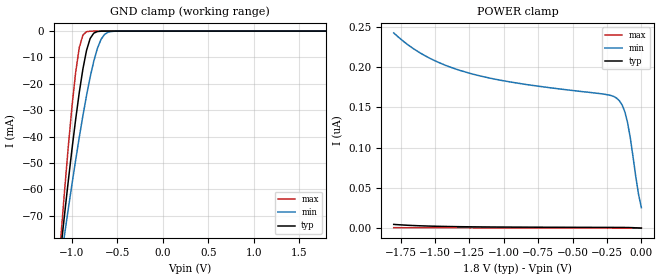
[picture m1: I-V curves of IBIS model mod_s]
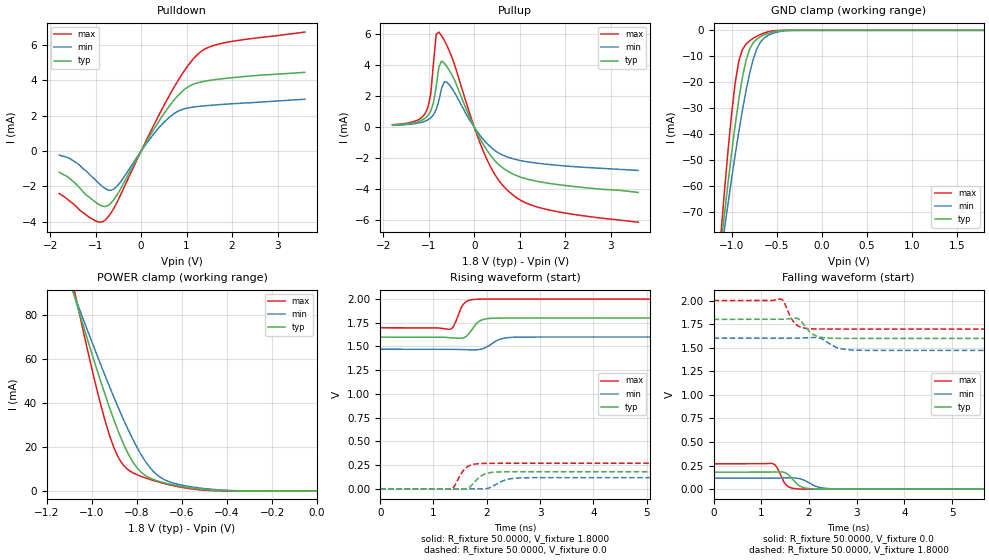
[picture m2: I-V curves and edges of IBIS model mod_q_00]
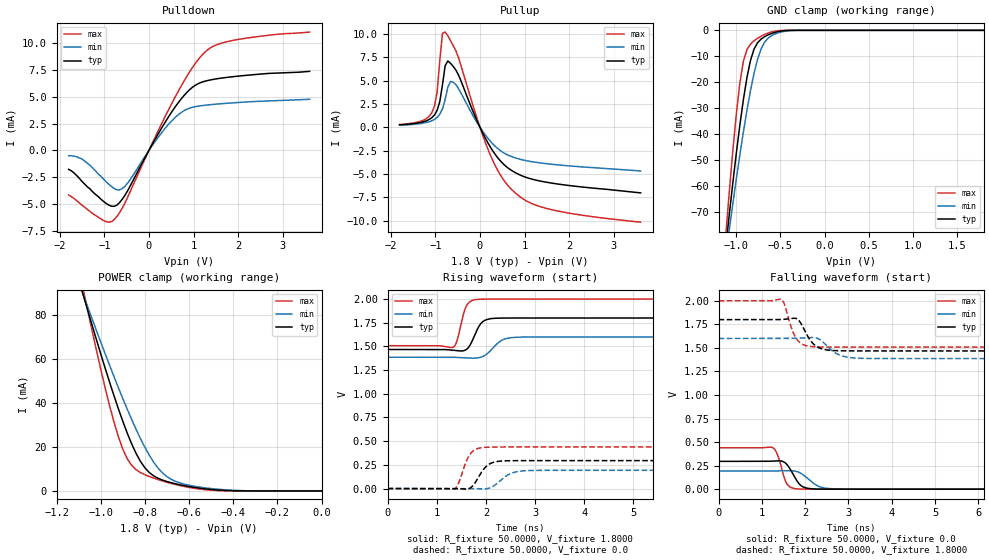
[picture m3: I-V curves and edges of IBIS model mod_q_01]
| IBIS file pin2_1v8_11.ibs created by s2ibis3 verion 1.1
| North Carolina State University, ERL, 2006
[IBIS ver]  4.0
[File name] pe_11_m95p32_1d8.ibs
[File Rev]  1.0
[Date]   18 Nov 2024
[Source]   CAD & Design Services (Catania) - STMicroelectronics
[Notes]
   (Note1)  This IBIS model includes the SO8N package parasitic data
   (Note2)  Pin 2 (S) and Pin 3,5,7 (WO2,DO0,HO3) have four driver
   stength cases: High, Medium, Qlow, Low;
   (Note3)  This IBIS model has some Notes about the non-monotonicity
   of the I-V curves, but they are not indicative of problems
   inside the model;
[Disclaimer]
   Customers are solely responsible for all aspects of their
   own product designs or applications using this IBIS Model.
   STMicroelectronics assumes no liability for Custmer Designs
   and applications associated to this IBIS Model.
   In the use of this IBIS Model Customer shall not modify,
   disassemble, alter this Model in whole or in part.
   If Customers do not accept these terms, the IBIS Model
   may not be used. For any problems or modifications please
   contact STMicroelectronics (www.st.com).
[Copyright] (c) 2024 STMicroelectronics
|   Component M95P32
[Component] M95P32
[Manufacturer] STMicroelectronics
[Package]
| variable  typ   min   max
R_pkg   0.0   0.0   0.0
L_pkg   0.0H   0.0H   0.0H
C_pkg   0.0F   0.0F   0.0F
[Pin]  signal_name   model_name   R_pin   L_pin   C_pin
1   S   mod_s   129.1m   2.1741nH   1.0266pF
2   QO1   mod_q   89.7m   1.6160nH   0.3359pF
3   WO2   mod_dwh   91.2m   1.6289nH   0.3576pF
4   VSS   GND   130.9m   2.1824nH   0.2874pF
5   DO0   mod_dwh   130.7m   2.1818nH   0.2862pF
6   C   mod_c   85.3m   1.5892nH   0.3544pF
7   HO3   mod_dwh   84.5m   1.5827nH   0.3547pF
8   VDD   POWER   124.1m   2.1422nH   0.2841pF
[Model Selector]   mod_q
mod_q_11   High drive: bit0='1', bit1='1'
mod_q_10   Med drive:  bit0='1', bit1='0'
mod_q_01   Qlow drive: bit0='0', bit1='1'
mod_q_00   Low drive:  bit0='0', bit1='0'
[Model Selector]   mod_dwh
mod_dwh_11   High drive: bit0='1', bit1='1'
mod_dwh_10   Med drive:  bit0='1', bit1='0'
mod_dwh_01   Qlow drive: bit0='0', bit1='1'
mod_dwh_00   Low drive:  bit0='0', bit1='0'
| Models and submodels in the file (10): mod_s (Input), mod_q_00 (Output), mod_q_01 (Output), mod_q_10 (Output), mod_q_11 (Output), mod_c (Input), mod_dwh_00 (I/O), mod_dwh_01 (I/O), mod_dwh_10 (I/O), mod_dwh_11 (I/O)
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|   Model mod_s
[Model]   mod_s
Model_type Input
Vinl   =   0.540V
Vinh   =   1.260V
C_comp   1.014pF   0.968pF   1.062pF
[Model Spec]
Vinl   0.540V  0.480V  0.600V  | <- for Vcc = 1.8V, 1.6V, 2.0V
Vinh   1.260V  1.120V  1.400V  | <- for Vcc = 1.8V, 1.6V, 2.0V
[Temperature Range]  25.0000   0.1050k   -40.0000
[Voltage Range]   1.8000V   1.6000V   2.0000V
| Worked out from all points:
|   GND clamp passes 1 mA (typ) near -0.76 V on its own axis
[GND_clamp]
|Voltage   I(typ)   I(min)   I(max)
-1.8V     -318.6mA   -262.3mA   -406.1mA
-1.12V    -81.69mA   -86.38mA   -77.02mA
-1.08V    -68.96mA   -76.72mA   -59.82mA
-1V       -44.75mA   -57.99mA   -28.59mA
-960mV    -33.58mA   -49mA      -15.76mA
-920mV    -23.34mA   -40.35mA   -6.304mA
-880mV    -14.41mA   -32.13mA   -1.515mA
-840mV    -7.357mA   -24.45mA   -241.6uA
-800mV    -2.808mA   -17.47mA   -33.89uA
-720mV    -178.3uA   -6.536mA   -639nA
-600mV    -1.717uA   -403.8uA   -1.818nA
1.8V      181.1pA    163.5nA    12.41pA
[POWER_clamp]
|Voltage   I(typ)   I(min)   I(max)
-1.8V     4.752nA    242.5nA    716.8pA
-1.6V     2.958nA    216.8nA    597.9pA
-1.3V     1.856nA    195nA      499.1pA
-940mV    1.384nA    181.2nA    411.6pA
-280mV    1.019nA    166.7nA    267.4pA
-180mV    972.8pA    161.5nA    245.7pA
-140mV    942.2pA    153.1nA    235.1pA
-120mV    914.3pA    144.4nA    228.4pA
-100mV    866.7pA    130.9nA    219.3pA
-80mV     784.6pA    111.7nA    205.6pA
-20mV     313.3pA    41.65nA    107.7pA
0V        181.1pA    25.55nA    69.35pA
|   Model mod_q_00
[Model]   mod_q_00
Model_type Output
Polarity   Non-Inverting
Enable   Active-High
Vmeas  =   0.900V
Cref   =   30.0pF
C_comp   1.630pF   1.607pF   1.683pF
[Model Spec]
Vmeas  0.900V  0.800V  1.000V  | <- for Vcc = 1.8V, 1.6V, 2.0V
[Temperature Range]  25.0000   0.1050k   -40.0000
[Voltage Range]   1.8000V   1.6000V   2.0000V
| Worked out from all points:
|   slope of the pulldown table from 0 to 0.27 V, typ, clamps not added: 227 ohm
|   slope of the pullup table from 0 to 0.27 V, typ, clamps not added: 188 ohm
|   GND clamp passes 1 mA (typ) near -0.58 V on its own axis
|   POWER clamp passes 1 mA (typ) near -0.53 V on its own axis
|   rising waveform, R_fixture 50.0000, V_fixture 1.8000: 20-80 % time 173ps typ, 233ps min, 138ps max; typ from 1.6 V to 1.8 V
|   rising waveform, R_fixture 50.0000, V_fixture 0.0: 20-80 % time 207ps typ, 255ps min, 179ps max; typ from 0 V to 0.18 V
|   falling waveform, R_fixture 50.0000, V_fixture 0.0: 20-80 % time 213ps typ, 282ps min, 161ps max; typ from 0.18 V to 0 V
|   falling waveform, R_fixture 50.0000, V_fixture 1.8000: 20-80 % time 224ps typ, 277ps min, 188ps max; typ from 1.8 V to 1.6 V
[Pulldown]
|Voltage   I(typ)   I(min)   I(max)
-1.8V     -1.2mA     -220uA     -2.4mA
-1.38V    -2mA       -730uA     -3.26mA
-1.02V    -2.85mA    -1.59mA    -3.92mA
-840mV    -3.125mA   -2.02mA    -3.993mA
-660mV    -2.931mA   -2.218mA   -3.494mA
-540mV    -2.525mA   -2.014mA   -2.958mA
240mV     1.064mA    846.5uA    1.267mA
660mV     2.681mA    2.001mA    3.324mA
960mV     3.505mA    2.404mA    4.584mA
1.26V     3.879mA    2.53mA     5.517mA
1.86V     4.122mA    2.659mA    6.148mA
3.6V      4.46mA     2.94mA     6.74mA
[Pullup]
|Voltage   I(typ)   I(min)   I(max)
-1.8V     160uA      130uA      180uA
-1.08V    602uA      410uA      907uA
-960mV    1.058mA    620uA      2.158mA
-900mV    1.592mA    816uA      4.119mA
-840mV    2.634mA    1.149mA    6.013mA
-780mV    3.914mA    1.734mA    6.153mA
-660mV    4.145mA    2.953mA    5.618mA
-600mV    3.902mA    2.912mA    5.267mA
180mV     -1.012mA   -717.7uA   -1.417mA
720mV     -2.795mA   -1.896mA   -4.031mA
1.5V      -3.538mA   -2.344mA   -5.223mA
3.6V      -4.19mA    -2.77mA    -6.11mA
[GND_clamp]
|Voltage   I(typ)   I(min)   I(max)
-1.8V     -319.7mA   -274.4mA   -407.3mA
-1.12V    -83.64mA   -87.01mA   -79.32mA
-1.08V    -71.08mA   -76.85mA   -62.45mA
-1V       -47.38mA   -57.28mA   -32.33mA
-960mV    -36.55mA   -47.99mA   -20.38mA
-920mV    -26.73mA   -39.15mA   -11.92mA
-840mV    -11.67mA   -23.32mA   -5.34mA
-760mV    -4.801mA   -11.23mA   -3.081mA
-720mV    -3.384mA   -7.183mA   -2.279mA
-640mV    -1.748mA   -2.99mA    -1.048mA
-440mV    -85.93uA   -314uA     -8.035uA
1.8V      367pA      1.678uA    95.55pA
[POWER_clamp]
|Voltage   I(typ)   I(min)   I(max)
-1.8V     354.3mA    299.2mA    462.7mA
-1.08V    89.41mA    89.52mA    92.12mA
-1.06V    82.53mA    84.01mA    82.65mA
-980mV    55.86mA    62.44mA    46.9mA
-920mV    37.35mA    46.96mA    24.63mA
-880mV    26.31mA    37.17mA    14.66mA
-840mV    17.07mA    28.03mA    9.669mA
-800mV    10.51mA    19.82mA    7.37mA
-740mV    5.731mA    10.32mA    5.151mA
-640mV    2.77mA     3.598mA    2.408mA
-420mV    154.7uA    391.9uA    29.01uA
0V        367pA      19.37nA    169pA
[Ramp]
| variable   typ   min   max
dV/dt_r  0.1078/0.2627n   70.1335m/0.3855n   0.1613/0.2256n
dV/dt_f  0.1212/0.3422n   77.4600m/0.5045n   0.1817/0.2879n
R_load = 50.0000
[Rising Waveform]
R_fixture= 50.0000
V_fixture= 1.8000
V_fixture_min= 1.6000
V_fixture_max= 2.0000
|time   V(typ)   V(min)   V(max)
0s        1.598V     1.471V     1.697V
1.312ns   1.593V     1.471V     1.682V
1.392ns   1.589V     1.469V     1.73V
1.504ns   1.587V     1.467V     1.89V
1.568ns   1.593V     1.466V     1.95V
1.792ns   1.732V     1.464V     1.997V
1.984ns   1.791V     1.491V     2V
2.24ns    1.799V     1.575V     2V
2.512ns   1.8V       1.598V     2V
8ns       1.8V       1.6V       2V
[Rising Waveform]
R_fixture= 50.0000
V_fixture= 0.0
V_fixture_min= 0.0
V_fixture_max= 0.0
|time   V(typ)   V(min)   V(max)
0s        6.626nV    816.4nV    1.089nV
1.336ns   88.47uV    172.2uV    -1.733mV
1.384ns   -220.2uV   182.8uV    20.7mV
1.528ns   -3.099mV   122.3uV    167.1mV
1.608ns   -1.582mV   -63.13uV   219.5mV
1.864ns   122.9mV    -2.68mV    265.2mV
2.088ns   172mV      19.92mV    268.4mV
2.344ns   179mV      91.64mV    268.8mV
2.632ns   179.7mV    114.2mV    268.8mV
8ns       179.7mV    116.9mV    268.8mV
[Falling Waveform]
R_fixture= 50.0000
V_fixture= 0.0
V_fixture_min= 0.0
V_fixture_max= 0.0
|time   V(typ)   V(min)   V(max)
0s        179.7mV    116.9mV    268.8mV
1.232ns   181.7mV    116.9mV    271.5mV
1.328ns   183.5mV    117.7mV    230.5mV
1.456ns   180.9mV    118.8mV    93.8mV
1.52ns    169.7mV    119.4mV    46.24mV
1.76ns    50.46mV    115.5mV    2.665mV
1.92ns    12.7mV     90.01mV    397.6uV
2.192ns   901uV      22.64mV    19.42uV
2.544ns   32.53uV    2.455mV    1.419uV
8ns       241.8nV    983nV      336.1nV
[Falling Waveform]
R_fixture= 50.0000
V_fixture= 1.8000
V_fixture_min= 1.6000
V_fixture_max= 2.0000
|time   V(typ)   V(min)   V(max)
0s        1.8V       1.6V       2V
1.424ns   1.8V       1.6V       2.013V
1.472ns   1.802V     1.6V       1.987V
1.696ns   1.812V     1.6V       1.762V
1.808ns   1.795V     1.602V     1.721V
2ns       1.677V     1.606V     1.701V
2.272ns   1.608V     1.593V     1.698V
2.592ns   1.599V     1.5V       1.697V
2.928ns   1.598V     1.474V     1.697V
8ns       1.598V     1.471V     1.697V
|   Model mod_q_01
[Model]   mod_q_01
Model_type Output
Polarity   Non-Inverting
Enable   Active-High
Vmeas  =   0.900V
Cref   =   30.0pF
C_comp   1.630pF   1.607pF   1.683pF
[Model Spec]
Vmeas  0.900V  0.800V  1.000V  | <- for Vcc = 1.8V, 1.6V, 2.0V
[Temperature Range]  25.0000   0.1050k   -40.0000
[Voltage Range]   1.8000V   1.6000V   2.0000V
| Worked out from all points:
|   slope of the pulldown table from 0 to 0.27 V, typ, clamps not added: 136 ohm
|   slope of the pullup table from 0 to 0.27 V, typ, clamps not added: 113 ohm
|   GND clamp passes 1 mA (typ) near -0.58 V on its own axis
|   POWER clamp passes 1 mA (typ) near -0.53 V on its own axis
|   rising waveform, R_fixture 50.0000, V_fixture 1.8000: 20-80 % time 187ps typ, 259ps min, 144ps max; typ from 1.47 V to 1.8 V
|   rising waveform, R_fixture 50.0000, V_fixture 0.0: 20-80 % time 234ps typ, 298ps min, 196ps max; typ from 0 V to 0.295 V
|   falling waveform, R_fixture 50.0000, V_fixture 0.0: 20-80 % time 236ps typ, 324ps min, 172ps max; typ from 0.295 V to 0 V
|   falling waveform, R_fixture 50.0000, V_fixture 1.8000: 20-80 % time 276ps typ, 347ps min, 223ps max; typ from 1.8 V to 1.47 V
[Pulldown]
|Voltage   I(typ)   I(min)   I(max)
-1.8V     -1.77mA    -500uA     -4.16mA
-1.5V     -2.9mA     -800uA     -5.12mA
-1.02V    -4.75mA    -2.66mA    -6.54mA
-840mV    -5.208mA   -3.37mA    -6.655mA
-660mV    -4.886mA   -3.696mA   -5.823mA
-540mV    -4.208mA   -3.356mA   -4.93mA
240mV     1.773mA    1.411mA    2.112mA
660mV     4.469mA    3.334mA    5.541mA
960mV     5.842mA    4.006mA    7.64mA
1.26V     6.464mA    4.216mA    9.195mA
1.92V     6.897mA    4.448mA    10.3mA
3.6V      7.38mA     4.77mA     11.05mA
[Pullup]
|Voltage   I(typ)   I(min)   I(max)
-1.8V     270uA      210uA      300uA
-1.08V    1.022mA    691uA      1.55mA
-960mV    1.813mA    1.051mA    3.765mA
-900mV    2.748mA    1.389mA    7.165mA
-840mV    4.548mA    1.964mA    10.06mA
-780mV    6.594mA    2.97mA     10.2mA
-660mV    6.854mA    4.91mA     9.291mA
-540mV    6.135mA    4.587mA    8.207mA
180mV     -1.687mA   -1.196mA   -2.362mA
720mV     -4.659mA   -3.16mA    -6.718mA
1.5V      -5.897mA   -3.906mA   -8.705mA
3.6V      -7.03mA    -4.68mA    -10.17mA
[GND_clamp]
|Voltage   I(typ)   I(min)   I(max)
-1.8V     -319.7mA   -274.4mA   -407.3mA
-1.12V    -83.64mA   -87.01mA   -79.32mA
-1.08V    -71.08mA   -76.85mA   -62.45mA
-1V       -47.38mA   -57.28mA   -32.33mA
-960mV    -36.55mA   -47.99mA   -20.38mA
-920mV    -26.73mA   -39.15mA   -11.92mA
-840mV    -11.67mA   -23.32mA   -5.34mA
-760mV    -4.801mA   -11.23mA   -3.081mA
-720mV    -3.384mA   -7.183mA   -2.279mA
-640mV    -1.748mA   -2.99mA    -1.048mA
-440mV    -85.93uA   -314uA     -8.035uA
1.8V      367pA      1.678uA    95.55pA
[POWER_clamp]
|Voltage   I(typ)   I(min)   I(max)
-1.8V     354.3mA    299.2mA    462.7mA
-1.08V    89.41mA    89.52mA    92.12mA
-1.06V    82.53mA    84.01mA    82.65mA
-980mV    55.86mA    62.44mA    46.9mA
-920mV    37.35mA    46.96mA    24.63mA
-880mV    26.31mA    37.17mA    14.66mA
-840mV    17.07mA    28.03mA    9.669mA
-800mV    10.51mA    19.82mA    7.37mA
-740mV    5.731mA    10.32mA    5.151mA
-640mV    2.77mA     3.598mA    2.408mA
-420mV    154.7uA    391.9uA    29.01uA
0V        367pA      12.25nA    169pA
[Ramp]
| variable   typ   min   max
dV/dt_r   0.1770/0.2926n   0.1156/0.4434n   0.2634/0.2414n
dV/dt_f   0.1994/0.4224n   0.1282/0.5939n   0.2952/0.3113n
R_load = 50.0000
[Rising Waveform]
R_fixture= 50.0000
V_fixture= 1.8000
V_fixture_min= 1.6000
V_fixture_max= 2.0000
|time   V(typ)   V(min)   V(max)
0s        1.468V     1.386V     1.508V
1.328ns   1.46V      1.386V     1.491V
1.408ns   1.455V     1.384V     1.555V
1.6ns     1.467V     1.379V     1.925V
1.808ns   1.661V     1.378V     1.996V
1.904ns   1.746V     1.387V     1.999V
2.016ns   1.783V     1.419V     2V
2.32ns    1.799V     1.564V     2V
2.592ns   1.8V       1.596V     2V
8ns       1.8V       1.6V       2V
[Rising Waveform]
R_fixture= 50.0000
V_fixture= 0.0
V_fixture_min= 0.0
V_fixture_max= 0.0
|time   V(typ)   V(min)   V(max)
0s        5.894nV    739nV      954.2pV
1.352ns   48.91uV    236.7uV    -5mV
1.432ns   -943.1uV   248.5uV    43.46mV
1.592ns   -5.481mV   17.62uV    277.8mV
1.672ns   3.071mV    -431.2uV   358.5mV
1.936ns   192.6mV    -4.139mV   433.1mV
2.184ns   281.3mV    37.23mV    438.4mV
2.488ns   294mV      154.8mV    438.9mV
2.792ns   294.9mV    188mV      438.9mV
8ns       295mV      192.6mV    438.9mV
[Falling Waveform]
R_fixture= 50.0000
V_fixture= 0.0
V_fixture_min= 0.0
V_fixture_max= 0.0
|time   V(typ)   V(min)   V(max)
0s        295mV      192.6mV    438.9mV
1.248ns   298.2mV    192.8mV    441.3mV
1.36ns    301mV      194mV      366.5mV
1.568ns   266.9mV    196.7mV    65.04mV
1.792ns   102mV      189.1mV    4.267mV
1.888ns   43.86mV    171.7mV    1.345mV
2.016ns   13.58mV    130.4mV    296.2uV
2.304ns   1.046mV    31.23mV    12.89uV
2.592ns   84.09uV    5.197mV    1.892uV
8ns       361.6nV    1.006uV    503.8nV
[Falling Waveform]
R_fixture= 50.0000
V_fixture= 1.8000
V_fixture_min= 1.6000
V_fixture_max= 2.0000
|time   V(typ)   V(min)   V(max)
0s        1.8V       1.6V       2V
1.464ns   1.801V     1.6V       2.01V
1.528ns   1.804V     1.6V       1.953V
1.784ns   1.813V     1.602V     1.608V
1.88ns    1.776V     1.604V     1.556V
2.104ns   1.59V      1.609V     1.516V
2.408ns   1.487V     1.564V     1.509V
2.744ns   1.47V      1.435V     1.508V
3.128ns   1.468V     1.393V     1.508V
8ns       1.468V     1.386V     1.508V
